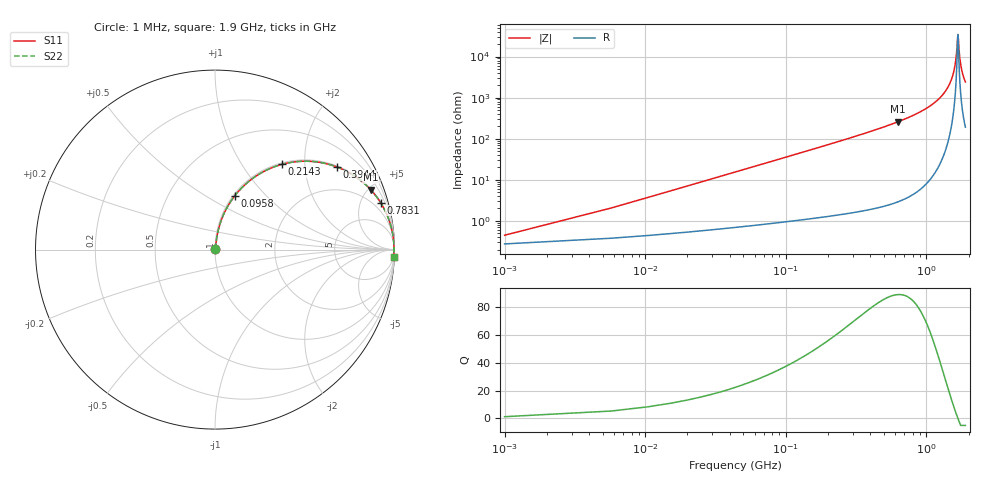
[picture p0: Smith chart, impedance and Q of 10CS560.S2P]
! Coilcraft 1008CS-560 Chip Inductor
! 02 July 2002
# MHZ S MA R 50
!Freq  MagS11  AngS11  MagS21  AngS21  MagS12  AngS12  MagS22  AngS22
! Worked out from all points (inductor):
!   402 points, 1 MHz to 1.9 GHz, reference 50 ohm
!   read as one part in series: L = 56 nH near 10.48 MHz
!   highest Q = 88.9 at 631.4 MHz (marker M1), where L = 65.2 nH
!   self-resonance near 1.679 GHz
!   S11 on the Smith chart (normalised r, x): 1 MHz: 1.01, +0.01; 95.8 MHz: 1.02, +0.68; 214.3 MHz: 1.03, +1.53; 394.4 MHz: 1.04, +2.94; 783.1 MHz: 1.08, +7.04; 1.9 GHz: 5, -48
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1  0.004447 51.9  0.9973 -0.2  0.9973 -0.2  0.004447 51.9
15.22  0.05344 81.7  0.9937 -3.1  0.9937 -3.1  0.05344 81.7
29.44  0.1026 80.8  0.9888 -5.9  0.9888 -5.9  0.1026 80.8
57.88  0.1985 76.4  0.9727 -11.4  0.9727 -11.4  0.1985 76.4
95.8  0.3178 69.9  0.9395 -18.5  0.9395 -18.5  0.3178 69.9
214.3  0.6034 51.9  0.7871 -37.1  0.7871 -37.1  0.6034 51.9
318.58  0.753 40.4  0.6476 -48.8  0.6476 -48.8  0.753 40.4
394.42  0.8217 34.0  0.5595 -55.3  0.5595 -55.3  0.8217 34.0
631.42  0.9292 21.1  0.3592 -68.3  0.3592 -68.3  0.9292 21.1
636.16  0.9304 20.9  0.3562 -68.5  0.3562 -68.5  0.9304 20.9
783.1  0.959 15.8  0.2725 -73.5  0.2725 -73.5  0.959 15.8
953.74  0.9776 11.4  0.1976 -77.8  0.1976 -77.8  0.9776 11.4
1271.32  0.993 5.5  0.09511 -83.1  0.09511 -83.1  0.993 5.5
1465.66  0.9963 2.7  0.04648 -84.2  0.04648 -84.2  0.9963 2.7
1584.16  0.9971 1.2  0.02029 -81.2  0.02029 -81.2  0.9971 1.2
1631.56  0.9972 0.6  0.01053 -74.1  0.01053 -74.1  0.9972 0.6
1674.22  0.9972 0.1  0.003198 -27.0  0.003198 -27.0  0.9972 0.1
1683.7  0.9971 -0.0  0.002897 8.8  0.002897 8.8  0.9971 -0.0
1726.36  0.997 -0.5  0.00935 71.2  0.00935 71.2  0.997 -0.5
1759.54  0.9969 -0.9  0.01558 78.1  0.01558 78.1  0.9969 -0.9
1821.16  0.9965 -1.5  0.02708 81.9  0.02708 81.9  0.9965 -1.5
1900  0.9959 -2.4  0.04135 83.1  0.04135 83.1  0.9959 -2.4
